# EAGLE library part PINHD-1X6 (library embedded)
PIN HEADER
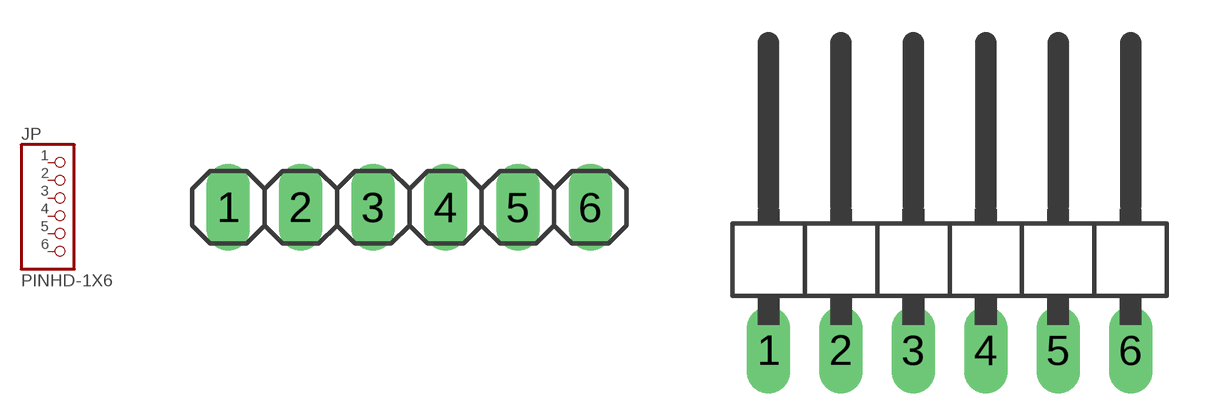
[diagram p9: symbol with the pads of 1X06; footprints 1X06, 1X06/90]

Designator prefix JP

## PINHD-1X6 (ANGLE: Straight; PACKAGE: Pin Header; PITCH: 2.54mm; POS: 6; ROWS: 1)  [1X06]
1  1  pas
2  2  pas
3  3  pas
4  4  pas
5  5  pas
6  6  pas

## PINHD-1X6/90 (ANGLE: 90; PACKAGE: Pin Header; PITCH: 2.54mm; POS: 6; ROWS: 1)  [1X06/90]
Pads as for 1X06

## Footprint 1X06 (pad centres in mm)
PIN HEADER
drill 1.016 long: 1 -6.35,0; 2 -3.81,0; 3 -1.27,0; 4 1.27,0; 5 3.81,0; 6 6.35,0

## Footprint 1X06/90 (pad centres in mm)
PIN HEADER
drill 1.016 long: 1 -6.35,-3.81; 2 -3.81,-3.81; 3 -1.27,-3.81; 4 1.27,-3.81; 5 3.81,-3.81; 6 6.35,-3.81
